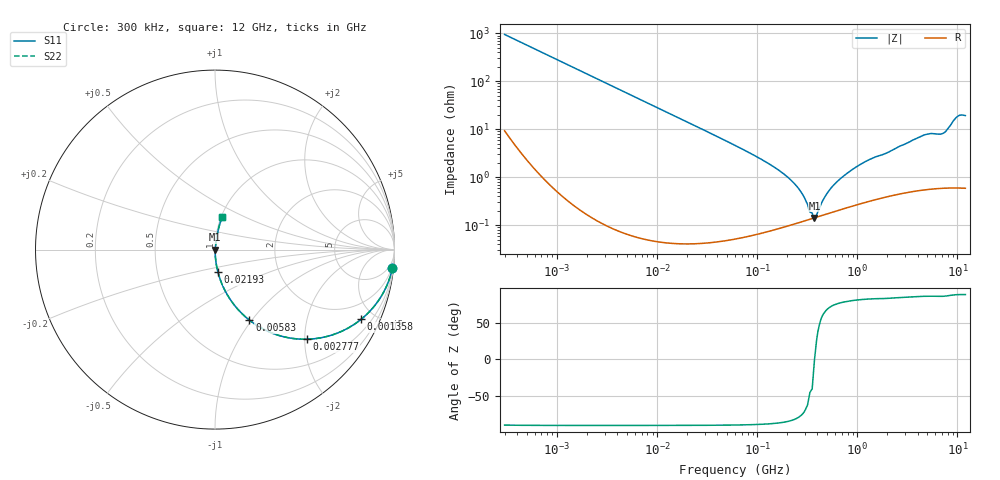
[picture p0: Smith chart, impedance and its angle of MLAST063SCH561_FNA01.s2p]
! MLAST063SCH561_FNA01  S-PARAMETER MODEL  ( General Type )
! Model Generated by TAIYO YUDEN Corporation (http://www.ty-top.com)
! Version 1.0
! TAIYO YUDEN Control No. 160830
! Copyright(c) 2016 TAIYO YUDEN CO.,LTD. All Rights Reserved.
! Product Description (link to TY-COMPAS)
! https://ds.yuden.co.jp/TYCOMPAS/or/detail?pn=MLAST063SCH561JFNA01&u=M
! Products Name : Multilayer Ceramic Capacitors
! Characteristics :
!  Capacitance : 560 pF , Rated Voltage : 25V , TCC : CH / C0H
!  Case Size : 0.6 x 0.3 / 0.024 x 0.012 [mm/inch] , Thickness : 0.3 / 0.012 [mm/inch]
!  (Conditions: Temperature = 25 degC , DC Bias Current/Voltage = 0A / 0V)
! External Node Assignments :
!  1  o---| |---o  2
! GND o---------o GND
! Frequency Range : 0.3MHz  -  12000MHz  [ 401 STEP ]
# MHz S RI R 50
! Freq[MHz].  S11 Real  S11 Imag  S21 Real  S21 Imag  S12 Real  S12 Imag  S22 Real  S22 Imag
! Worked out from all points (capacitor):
!   401 points, 300 kHz to 12 GHz, reference 50 ohm
!   read as one part in series: C = 560 pF near 316.3 kHz
!   lowest |Z| = 142 mohm at 373.3 MHz (marker M1)
!   series resonance near 373.5 MHz, so ESL is about 320 pH
!   S11 on the Smith chart (normalised r, x): 300 kHz: 1, -19; 1.358 MHz: 1.01, -4.19; 2.777 MHz: 1.00, -2.05; 5.83 MHz: 1.00, -0.97; 21.93 MHz: 1.00, -0.26; 12 GHz: 1.01, +0.39
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0.3  0.988 -0.1042  0.012 0.1042  0.012 0.1042  0.988 -0.1042
0.719103  0.9393 -0.2375  0.0607 0.2375  0.0607 0.2375  0.9393 -0.2375
1.358047  0.8138 -0.3886  0.1862 0.3886  0.1862 0.3886  0.8138 -0.3886
1.769972  0.7203 -0.4483  0.2797 0.4483  0.2797 0.4483  0.7203 -0.4483
2.776859  0.5116 -0.4993  0.4884 0.4993  0.4884 0.4993  0.5116 -0.4993
5.830396  0.1922 -0.3934  0.8078 0.3934  0.8078 0.3934  0.1922 -0.3934
10.44266  0.0692 -0.253  0.9308 0.253  0.9308 0.253  0.0692 -0.253
21.92581  0.0168 -0.127  0.9832 0.127  0.9832 0.127  0.0168 -0.127
60  0.00263 -0.046  0.9974 0.046  0.9974 0.046  0.00263 -0.046
129.3602  0.00111 -0.0193  0.9989 0.0193  0.9989 0.0193  0.00111 -0.0193
208.3979  0.00107 -0.00937  0.9989 0.00937  0.9989 0.00937  0.00107 -0.00937
278.9009  0.0012 -0.00449  0.9988 0.00449  0.9988 0.00449  0.0012 -0.00449
353.9943  0.00137 -0.00115  0.9986 0.00115  0.9986 0.00115  0.00137 -0.00115
373.2558  0.00142 -9.95e-06  0.9986 9.95e-06  0.9986 9.95e-06  0.00142 -9.95e-06
512.9422  0.00177 0.00467  0.9982 -0.00467  0.9982 -0.00467  0.00177 0.00467
686.4755  0.00219 0.00927  0.9978 -0.00927  0.9978 -0.00927  0.00219 0.00927
1166.079  0.00333 0.0201  0.9967 -0.0201  0.9967 -0.0201  0.00333 0.0201
2088.533  0.00512 0.0335  0.9949 -0.0335  0.9949 -0.0335  0.00512 0.0335
4623.766  0.011 0.0744  0.989 -0.0744  0.989 -0.0744  0.011 0.0744
7064.448  0.0122 0.0794  0.9878 -0.0794  0.9878 -0.0794  0.0122 0.0794
9968.853  0.038 0.1757  0.962 -0.1757  0.962 -0.1757  0.038 0.1757
12000  0.041 0.1837  0.959 -0.1837  0.959 -0.1837  0.041 0.1837
